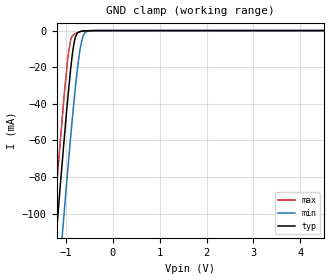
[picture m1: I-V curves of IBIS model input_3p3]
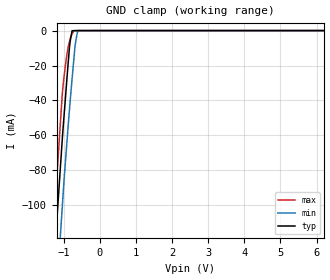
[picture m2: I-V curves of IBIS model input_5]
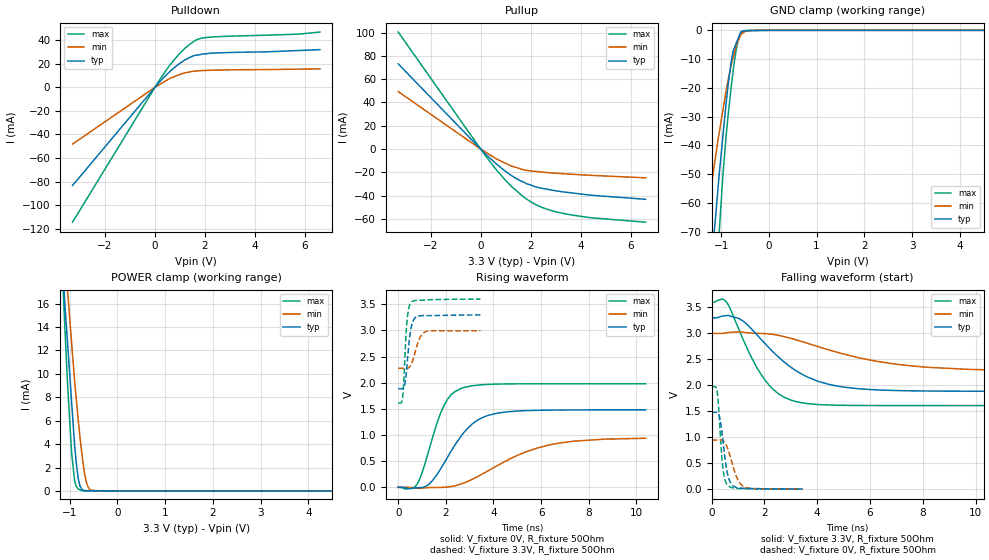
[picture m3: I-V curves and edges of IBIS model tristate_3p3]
|Texas Instruments Incorporated
| 2.35V-5.25V, 10 Bit, 1.25MSPS, Serial ADC
| Marketing part#   Digital Voltage Range   Package-type   #pins
| ADS7887SDBVR   2.35V - 5.25V   SOT-23   6
| ADS7887SDBVT   2.35V - 5.25V   SOT-23   6
| ADS7887SDBVTG4   2.35V - 5.25V   SOT-23   6
| ADS7887SDCKR   2.35V - 5.25V   SC70   6
| ADS7887SDCKT   2.35V - 5.25V   SC70   6
| ADS7887SDCKTG4   2.35V - 5.25V   SC70   6
[IBIS Ver]   3.2
[File name]   ads7887.ibs
|SIMDE Ver   V3.0 - 201101 - RHL4 - Build 450
[File Rev]   1.0
[Date]   4/14/2011
[Source]
| Texas Instruments Incorporated.
| Analog-eLab Design Center, HPA
| 12500 TI Blvd
| Dallas, TX -75243
| e-mail: elab_ibis@list.ti.com
| -Model generated from simulations in TISPICE
[Notes]   Revision History:
| Rev 1.0: 4/14/2011
| - Initial version of the model
| - Model generated from simulations in TISPICE
| - Model matched to SPICE simulation
| - C_comp although listed in numerical order of value are
|   obtained from varying PVT conditions. For PVT conditions for
|   each specific value refer the buffer description under
|   respective [Model]. IBIS model user is responsible for using
|   appropriate C_comp to simulate for Signal Integrity.
| - Model names with a trailing _3p3 contains
|   the model for 3.3V [3.0V and 3.6V]. Model names with trailing _5
|   contains the model for 5.0V [4.75V and 5.25V] operation.
[Disclaimer]
| This model is designed as an aid for customers of Texas Instruments.
| TI and its licensors and suppliers make no warranties, either expressed
| or implied, with respect to this  model, including the warranties of
| merchantability or fitness for a particular purpose. The model is
| provided solely on an "as is" basis. The entire risk as to its quality
| and performance is with the customer.
[Copyright]
 (C) Copyright 2011 Texas Instruments Incorporated.All rights reserved.
|   ADS7887DCK
[Component]   ADS7887DCK
[Manufacturer]   TI
[Package]   |6 SC70   -  DCK package
|   typ   min   max
R_pkg   0.00702   0.00692   0.00708
L_pkg   0.97194nH   0.95184nH   0.98458nH
C_pkg   0.21320pF   0.20251pF   0.24324pF
[Pin]  signal_name   model_name   R_pin   L_pin   C_pin
1   VDD   POWER   0.00686   0.95373nH  0.21120pF
2   GND   GND   0.00692   0.90692nH  0.21786pF
3   VIN   TERM   0.00707   0.98458nH  0.20251pF
4   SCLK   SCLK_CS   0.00701   0.97148nH  0.20453pF
5   SDO   SDO   0.00692   0.95184nH  0.24324pF
6   _CS   SCLK_CS   0.00708   0.97988nH  0.20253pF
|   ADS7887DBV
[Component]   ADS7887DBV
[Manufacturer]   TI
[Package]   |6 SOT23  -  DBV package
|   typ   min   max
R_pkg   0.00702   0.00692   0.00708
L_pkg   0.97194nH   0.95184nH   0.98458nH
C_pkg   0.21320pF   0.20251pF   0.24324pF
[Pin]  signal_name   model_name   R_pin   L_pin   C_pin
1   VDD   POWER   0.00686   0.95373nH  0.21120pF
2   GND   GND   0.00692   0.90692nH  0.21786pF
3   VIN   TERM   0.00707   0.98458nH  0.20251pF
4   SCLK   SCLK_CS   0.00701   0.97148nH  0.20453pF
5   SDO   SDO   0.00692   0.95184nH  0.24324pF
6   _CS   SCLK_CS   0.00708   0.97988nH  0.20253pF
|   Model Selectors
[Model Selector] SCLK_CS
input_3p3  3.3V digital input
input_5   5.0V digital input
[Model Selector] SDO
tristate_3p3  3.3V digital 3-state
tristate_5   5.0V digital 3-state
[Model Selector] TERM
term_3-3V  3.3V nominal termination
term_5-0V  5.0V nominal termination
[Model]  term_3-3V
Model_type Terminator
C_comp   1.0e-20F  1.0e-20F  1.0e-20F
|   typ   min   max
[Voltage Range]   3.3V   3.0V   3.6V
[POWER Clamp Reference]   3.3V   3.0V   3.6V
[GND Clamp Reference]   0V   0V   0V
|Ambient Temperature   25   125   -40
|Junction Temperature
[Temperature Range]   28   128   -40
[Model]  term_5-0V
Model_type Terminator
C_comp   1.0e-20F  1.0e-20F  1.0e-20F
|   typ   min   max
[Voltage Range]   5.0V   4.75V   5.25V
[POWER Clamp Reference]   5.0V   4.75V   5.25V
[GND Clamp Reference]   0V   0V   0V
|Ambient Temperature   25   125   -40
|Junction Temperature
[Temperature Range]   28   128   -40
| Models and submodels in the file (6): input_3p3 (Input), input_5 (Input), tristate_3p3 (3-state), tristate_5 (3-state), term_3-3V (Terminator), term_5-0V (Terminator)
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|   input_3p3 Model
[Model]   input_3p3
Model_type   Input
Vinl = 0.4
Vinh = 2.9
|   typ   min   max
|   (nom PVT)   (Fast PVT)   (slow PVT)
|C_comp from frequency method(F=25MHz)
|Average
|C_comp   5.239e-13   3.992e-13   6.559e-13
|C_comp from L-C Tank method(L=1nH)
|Resonant Frequency(Hz)   1.025e10   1.197e10   9.050e09
C_comp   2.413e-13   1.770e-13   3.096e-13
| Where nom  PVT is Nominal Process,  3.3V,  28C
|   Fast PVT is Strong Process,   3.6V,  -40C
|   Slow PVT is Weak Process,   3V,  128C
[Model spec]
Vinh   2.90   2.60   3.20
[Voltage Range]   3.3   3   3.6
|Ambient Temperature   25   125   -40
|Junction Temperature
[Temperature Range]   28   128   -40
[Power Clamp Reference]   3.3   3   3.6
[GND Clamp Reference]   0   0   0
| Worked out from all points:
|   GND clamp passes 1 mA (typ) near -0.74 V on its own axis
[GND Clamp]
|   Voltage   I(typ)   I(min)   I(max)
-3.3V     -822.3mA   -852.6mA   -804.8mA
-1.29V    -139.2mA   -179.7mA   -115.4mA
-1.167V   -99.75mA   -139.8mA   -75.12mA
-1.112V   -82.19mA   -122.7mA   -58.28mA
-1.037V   -59.47mA   -99.28mA   -35.2mA
-954mV    -35.64mA   -74.23mA   -13.76mA
-896.4mV  -20.35mA   -57.53mA   -4.773mA
-806.4mV  -4.6mA     -33.27mA   -1.7mA
-744mV    -1.093mA   -18.76mA   -1.084mA
-669mV    -292.1uA   -6.315mA   -455.1uA
-540mV    -136.1uA   -341.1uA   -33.26uA
6.6V      0A         0A         0A
[POWER Clamp]
|   Voltage   I(typ)   I(min)   I(max)
-3.3V     0A         0A         0A
0V        0A         0A         0A
6.6V      0A         0A         0A
|   input_5 Model
[Model]   input_5
Model_type   Input
Vinl = 0.8
Vinh = 4.6
|   typ   min   max
|   (nom PVT)   (Fast PVT)   (slow PVT)
|C_comp from frequency method(F=25MHz)
|Average
|C_comp   4.762e-13   3.682e-13   5.878e-13
|C_comp from L-C Tank method(L=1nH)
|Resonant Frequency(Hz)   1.069e10   1.233e10   9.520e09
C_comp   2.219e-13   1.668e-13   2.798e-13
| Where nom  PVT is Nominal Process,  5V,  28C
|   Fast PVT is Strong Process,   5.25V,  -40C
|   Slow PVT is Weak Process,   4.75V,  128C
[Model spec]
Vinh   4.6   4.35   4.85
[Voltage Range]   5   4.75   5.25
|Ambient Temperature   25   125   -40
|Junction Temperature
[Temperature Range]   28   128   -40
[Power Clamp Reference]   5   4.75   5.25
[GND Clamp Reference]   0   0   0
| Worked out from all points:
|   GND clamp passes 1 mA (typ) near -0.78 V on its own axis
[GND Clamp]
|   Voltage   I(typ)   I(min)   I(max)
-5V       -1.408A    -1.434A    -1.395A
-1.341V   -156mA     -195.7mA   -131.8mA
-1.246V   -125.2mA   -165.1mA   -101.2mA
-1.042V   -62.47mA   -101.1mA   -36.63mA
-994.2mV  -49.49mA   -86.34mA   -26.73mA
-936.5mV  -33.99mA   -70.37mA   -17.06mA
-868.2mV  -16.28mA   -52mA      -8.526mA
-840mV    -9.204mA   -44.86mA   -6.185mA
-770mV    -93.47uA   -27.75mA   -2.019mA
-687mV    -44.98uA   -8.718mA   -33.21uA
-611mV    -584.2nA   -111uA     0A
10V       0A         0A         0A
[POWER Clamp]
|   Voltage   I(typ)   I(min)   I(max)
-5V       0A         0A         0A
0V        0A         0A         0A
10V       0A         0A         0A
|   tristate_3p3 Model
[Model]   tristate_3p3
Model_type   3-state
Polarity   Non-Inverting
Vmeas = 1.65
Vref  = 1.65
Cref  = 50pF
Rref  = 50
|   typ   min   max
|   (nom PVT)   (Fast PVT)   (slow PVT)
|C_comp from frequency method(F=25MHz)
|Average
|C_comp   4.760e-12   3.737e-12   6.048e-12
|ON state : BUFFER OUTPUT TURNED HIGH
|C_comp   4.760e-12   3.737e-12   6.048e-12
|OFF state: BUFFER IN HIGH IMPEDANCE
|C_comp   2.654e-12   1.944e-12   3.210e-12
|C_comp from L-C Tank method(L=1nH)
C_comp   2.046e-12   1.561e-12   2.572e-12
|ON state : BUFFER OUTPUT TURNED HIGH
|Resonant Frequency(Hz)   3.520e09   4.030e09   3.140e09
|C_comp   2.046e-12   1.561e-12   2.572e-12
|OFF state: BUFFER IN HIGH IMPEDANCE
|Resonant Frequency(Hz)   3.560e09   4.110e09   3.180e09
|C_comp   2.001e-12   1.501e-12   2.507e-12
| Where nom  PVT is Nominal Process,  3.3V,  28C
|   Fast PVT is Strong Process,   3.6V,  -40C
|   Slow PVT is Weak Process,   3V,  128C
[Voltage Range]   3.3   3   3.6
|Ambient Temperature   25   125   -40
|Junction Temperature
[Temperature Range]   28   128   -40
[Pullup Reference]   3.3   3   3.6
[Pulldown Reference]   0   0   0
[Power Clamp Reference]   3.3   3   3.6
[GND Clamp Reference]   0   0   0
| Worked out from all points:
|   slope of the pulldown table from 0 to 0.495 V, typ, clamps not added: 43.8 ohm
|   slope of the pullup table from 0 to 0.495 V, typ, clamps not added: 48.6 ohm
|   GND clamp passes 1 mA (typ) near -0.60 V on its own axis
|   POWER clamp passes 1 mA (typ) near -0.82 V on its own axis
|   falling waveform, V_fixture 3.3V, R_fixture 50Ohm: 20-80 % time 1.96ns typ, 3.45ns min, 1.24ns max; typ from 3.3 V to 1.89 V
|   rising waveform, V_fixture 0V, R_fixture 50Ohm: 20-80 % time 1.34ns typ, 2.57ns min, 864ps max; typ from 0 V to 1.48 V
|   rising waveform, V_fixture 3.3V, R_fixture 50Ohm: 20-80 % time 191ps typ, 299ps min, 142ps max; typ from 1.89 V to 3.3 V
|   falling waveform, V_fixture 0V, R_fixture 50Ohm: 20-80 % time 231ps typ, 361ps min, 165ps max; typ from 1.48 V to 0.005 V
[Pulldown]
|   Voltage   I(typ)   I(min)   I(max)
-3.3V     -83.41mA   -48.26mA   -114.5mA
172.8mV   4.268mA    2.197mA    5.912mA
662.4mV   14.71mA    8.083mA    20.63mA
939.6mV   19.51mA    10.44mA    27.58mA
1.246V    23.77mA    12.39mA    34.04mA
1.588V    27.03mA    13.72mA    39.51mA
2.012V    28.36mA    14.29mA    42.16mA
5.774V    31.23mA    15.41mA    45.16mA
6.6V      31.95mA    15.64mA    46.85mA
[GND Clamp]
|   Voltage   I(typ)   I(min)   I(max)
-3.3V     -556.1mA   -361.6mA   -764.2mA
-1.375V   -117.1mA   -74.77mA   -167.7mA
-1.278V   -96.95mA   -62.51mA   -138.5mA
-1.208V   -82.45mA   -54.42mA   -118.2mA
-1.074V   -56.71mA   -39.05mA   -79.52mA
-1.036V   -49.43mA   -35.23mA   -69.24mA
-896.4mV  -25.5mA    -21.12mA   -36.84mA
-781.2mV  -10.29mA   -11.52mA   -18.62mA
-745.8mV  -7.085mA   -9.26mA    -13.87mA
-651.6mV  -3.158mA   -3.938mA   -4.049mA
-541.2mV  -198.1uA   -878.6uA   -359.1uA
6.6V      0A         0A         0A
[Pullup]
|   Voltage   I(typ)   I(min)   I(max)
-3.3V     73.11mA    49.34mA    100.4mA
0V        0A         0A         0A
478.8mV   -9.863mA   -6.393mA   -13.81mA
1.188V    -22.06mA   -14.16mA   -31.08mA
1.706V    -28.18mA   -17.7mA    -40.89mA
1.818V    -29.64mA   -18.2mA    -42.59mA
2.239V    -32.57mA   -19.25mA   -48.04mA
3.089V    -36.06mA   -20.79mA   -54.2mA
4.497V    -39.7mA    -22.6mA    -59.06mA
6.6V      -43.05mA   -24.65mA   -62.7mA
[POWER Clamp]
|   Voltage   I(typ)   I(min)   I(max)
-3.3V     137.8mA    118mA      160.6mA
-1.782V   63.16mA    55.4mA     73.51mA
-1.102V   16.02mA    20.05mA    14.09mA
-1.048V   12.79mA    17.21mA    9.343mA
-961.2mV  7.672mA    12.72mA    3.298mA
-896.4mV  3.856mA    9.354mA    842.9uA
-858mV    2.212mA    7.641mA    384.2uA
-818.4mV  991.4uA    5.963mA    165.7uA
-774mV    341.6uA    4.191mA    54.51uA
-666mV    22.4uA     1.007mA    2.338uA
-549mV    18.45uA    58.44uA    427.5nA
6.6V      0A         0A         0A
[Ramp]
R_load = 50
|   typ   min   max
dV/dt_r   0.889339/1.34262e-09   0.568019/2.61473e-09   1.18777/8.6258e-10
dV/dt_f   0.849076/1.96215e-09   0.434704/3.4589e-09   1.19342/1.23869e-09
[Falling Waveform]
V_fixture = 3.3V
V_fixture_min = 3V
V_fixture_max = 3.6V
R_fixture = 50Ohm
|   Time   V(typ)   V(min)   V(max)
0s        3.3V       3V         3.6V
410ps     3.333V     3.002V     3.661V
583ps     3.345V     3.013V     3.591V
1.232ns   3.222V     3.021V     2.841V
2.012ns   2.811V     2.997V     2.11V
2.571ns   2.528V     2.959V     1.827V
3.16ns    2.295V     2.883V     1.693V
4.751ns   1.987V     2.638V     1.618V
7.547ns   1.895V     2.376V     1.611V
14.57ns   1.885V     2.278V     1.611V
[Rising Waveform]
V_fixture = 0V
V_fixture_min = 0V
V_fixture_max = 0V
R_fixture = 50Ohm
|   Time   V(typ)   V(min)   V(max)
0s        1.015nV    1.756nV    912pV
786ps     -8.352mV   -16.7mV    55.57mV
1.299ns   63.99mV    -5.506mV   726.5mV
1.911ns   451.1mV    -202.4uV   1.55V
2.269ns   727.5mV    18.47mV    1.791V
2.669ns   997.2mV    68.68mV    1.896V
3.213ns   1.248V     176.3mV    1.947V
3.777ns   1.376V     315.6mV    1.967V
6.309ns   1.475V     806.1mV    1.979V
10.39ns   1.481V     937.8mV    1.98V
[Rising Waveform]
V_fixture = 3.3V
V_fixture_min = 3V
V_fixture_max = 3.6V
R_fixture = 50Ohm
|   Time   V(typ)   V(min)   V(max)
0s        1.885V     2.275V     1.611V
177ps     1.885V     2.275V     1.688V
226ps     1.9V       2.275V     1.966V
275ps     1.971V     2.275V     2.44V
369ps     2.332V     2.275V     3.181V
533ps     3.032V     2.342V     3.532V
666ps     3.218V     2.511V     3.568V
879ps     3.277V     2.83V      3.575V
1.171ns   3.283V     2.98V      3.582V
3.453ns   3.296V     2.993V     3.599V
[Falling Waveform]
V_fixture = 0V
V_fixture_min = 0V
V_fixture_max = 0V
R_fixture = 50Ohm
|   Time   V(typ)   V(min)   V(max)
0s        1.481V     947.3mV    1.976V
162ps     1.481V     947mV      1.968V
217ps     1.479V     947.1mV    1.864V
304ps     1.395V     948.3mV    1.286V
415ps     1.003V     941mV      470.5mV
489ps     676.6mV    910.2mV    221.2mV
605ps     294.1mV    790.5mV    78.64mV
805ps     70.62mV    455.9mV    26.93mV
1.187ns   19.16mV    62.61mV    11.47mV
3.452ns   4.898mV    7.246mV    2.053mV
